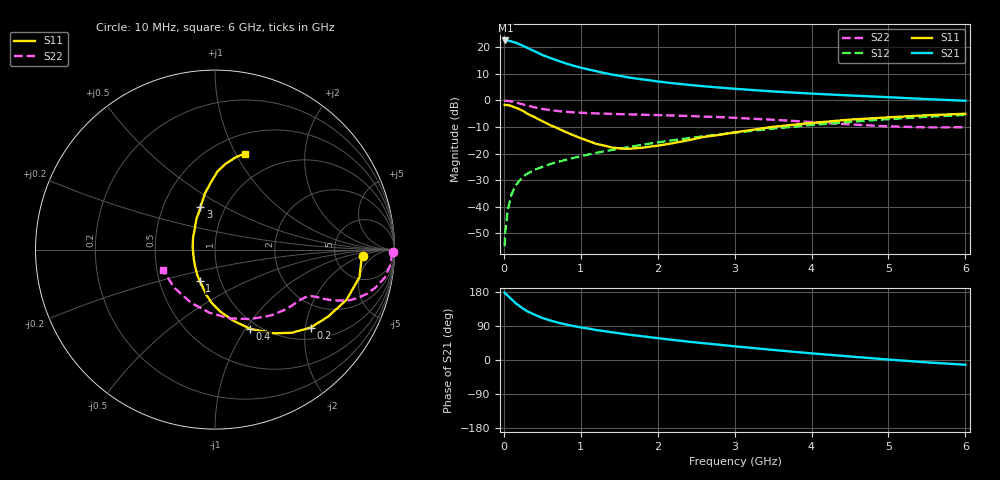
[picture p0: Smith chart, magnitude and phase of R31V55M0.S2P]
! SIEMENS Small Signal Semiconductors
! BFR181
! Si NPN RF Bipolar Junction Transistor in SOT23
! VCE = 1.5 V  IC = 5 mA
! Common Emitter S-Parameters:  May  1996
# GHz  S  MA  R  50
!  f  S11  S21  S12  S22
! GHz  MAG  ANG  MAG  ANG  MAG  ANG  MAG  ANG
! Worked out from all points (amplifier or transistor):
!   36 points, 10 MHz to 6 GHz, reference 50 ohm
!   highest |S21| = 22.6 dB at 20 MHz (marker M1)
!   |S21| within 3 dB of that: start of sweep to 321.5 MHz
!   unconditionally stable (mu >= 1): 999.2 MHz to 3.008 GHz
!   at 250 MHz: K = 0.43, MSG = 24.7 dB, |S12| = -28.8 dB
!   at 1.4 GHz: K = 1.07, MAG = 12.7 dB, |S12| = -18.7 dB
!   at 6 GHz: K = 0.87, MSG = 2.7 dB, |S12| = -5.5 dB
!   S11 on the Smith chart (normalised r, x): 10 MHz: 10, -2; 200 MHz: 1.30, -2.14; 400 MHz: 0.91, -1.05; 1 GHz: 0.80, -0.29; 3 GHz: 0.77, +0.39; 6 GHz: 0.70, +1.09
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0.01  0.8237 -2.3  13.44 178.0  0.0018 94.6  0.991 -0.9
0.02  0.8176 -4.5  13.47 175.7  0.0034 85.4  0.9852 -2.0
0.05  0.8194 -10.9  13.4 169.8  0.0086 84.1  0.9809 -4.9
0.1  0.784 -21.0  12.9 160.4  0.017 79.1  0.9596 -9.3
0.15  0.7322 -30.7  12.3 150.4  0.0244 74.3  0.919 -13.3
0.2  0.6876 -39.2  11.48 142.8  0.0305 70.4  0.8799 -16.3
0.25  0.6305 -47.3  10.64 135.5  0.0364 67.6  0.8407 -18.7
0.3  0.5707 -54.8  9.866 129.1  0.0414 65.5  0.8034 -20.5
0.4  0.4838 -66.0  8.424 119.5  0.0494 63.2  0.7393 -22.6
0.5  0.4064 -75.9  7.195 111.1  0.056 62.3  0.692 -23.8
0.6  0.3446 -85.5  6.33 104.5  0.0632 61.8  0.6588 -24.5
0.7  0.2983 -93.4  5.62 98.9  0.0692 62.0  0.6325 -24.9
0.8  0.256 -101.1  5.009 94.0  0.0758 62.0  0.6127 -25.3
1  0.1943 -116.1  4.146 86.1  0.0887 62.8  0.5868 -26.3
1.1  0.1724 -125.0  3.832 82.8  0.0958 63.3  0.5786 -26.9
1.6  0.1227 -177.3  2.745 67.5  0.1312 63.6  0.5478 -31.3
2.2  0.1569 136.6  2.103 53.0  0.178 62.1  0.5199 -38.8
3  0.2497 108.9  1.657 36.1  0.2474 57.3  0.4708 -52.1
3.5  0.3188 100.1  1.475 26.6  0.2945 53.2  0.4326 -63.5
4.5  0.435 88.2  1.239 9.3  0.3944 42.5  0.3533 -95.0
5.5  0.526 77.5  1.059 -6.2  0.4912 29.5  0.3108 -136.4
6  0.5609 72.6  0.985 -12.6  0.5336 22.4  0.3124 -158.4
